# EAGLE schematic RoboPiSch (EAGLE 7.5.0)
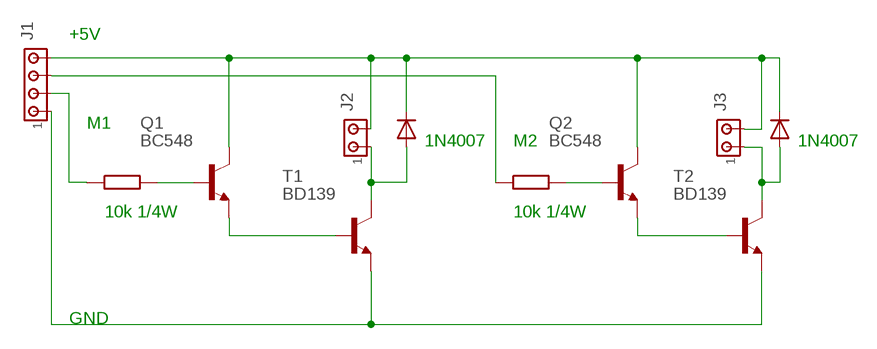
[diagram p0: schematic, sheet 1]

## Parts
J1  MTA04-100  [10X04MTA]
J2  MTA02-100  [10X02MTA]
J3  MTA02-100  [10X02MTA]
Q1  BC548  [TO92-EBC]
Q2  BC548  [TO92-EBC]
T1  BD139  [TO126]
T2  BD139  [TO126]

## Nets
N$1: Q1.B
N$2: Q1.E T1.3(B)
N$3: Q2.B
N$4: Q2.E T2.3(B)
N$5: J1.4 J2.2 J3.2 Q1.C Q2.C
N$7: J1.1 T1.1(E) T2.1(E)
N$8: J1.2
N$9: J1.3
N$10: J2.1 T1.2(C)
N$11: J3.1 T2.2(C)

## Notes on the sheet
- +5V
- M1
- 1N4007 | M2 | 1N4007
- 10k 1/4W | 10k 1/4W
- GND

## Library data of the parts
J1 = con-amp:MTA04-100: AMP connector
J2 J3 = con-amp:MTA02-100: AMP connector
Q1 Q2 = transistor-npn:BC548*: NPN Transistor
T1 T2 = transistor:BD139: NPN TRANSISTOR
